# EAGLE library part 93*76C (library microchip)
8K Microwire Compatible Serial EEPROM Source: http://ww1.microchip.com/downloads/en/DeviceDoc/21796H.pdf
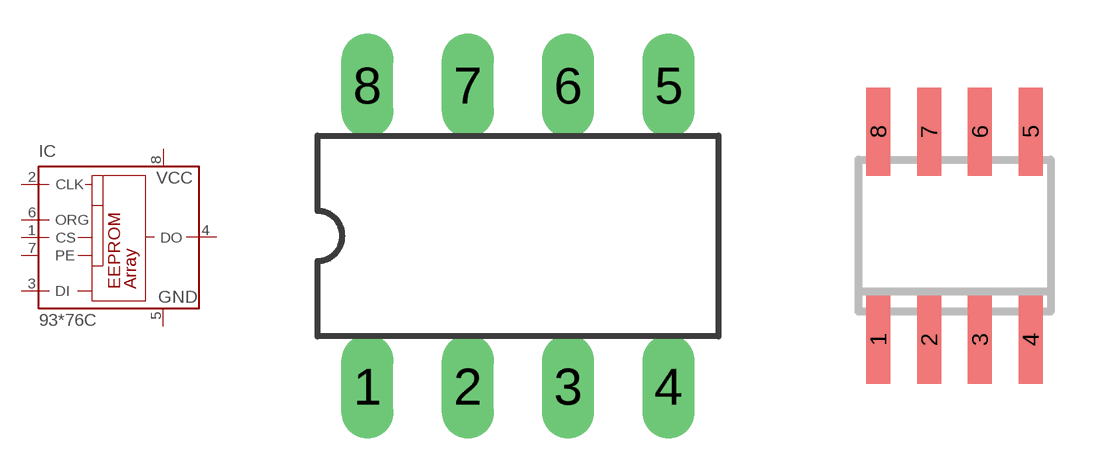
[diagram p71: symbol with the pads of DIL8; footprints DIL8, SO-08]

Designator prefix IC

## 93AA76CP (MF: MICROCHIP; MPN: 93AA76C-I/P; OC_FARNELL: 1331446; OC_NEWARK: 61H6457), 93C76CP (MF: MICROCHIP; MPN: 93C76C-I/P; OC_FARNELL: unknown; OC_NEWARK: 61H6696), 93LC76CP (MPN: 93LC76C-I/P; OC_FARNELL: 1556171; OC_NEWARK: 95M3420)  [DIL8]
1  CS  in
2  CLK  in
3  DI  in
4  DO  hiz
5  GND  pwr
6  ORG  in
7  PE  in
8  VCC  pwr

## 93AA76CSN (MPN: 93AA76C-I/SN; OC_FARNELL: 1331447; OC_NEWARK: 35M2485), 93C76CSN (MF: MICROCHIP; MPN: 93C76C-I/SN; OC_FARNELL: 1815963; OC_NEWARK: 61H6698), 93LC76CSN (MF: MICROCHIP; MPN: 93LC76C-I/SN; OC_FARNELL: unknown; OC_NEWARK: 96K4113)  [SO-08]
Pads as for DIL8

## 93AA76CST (MF: MICROCHIP; MPN: 93AA76CT-I/ST; OC_FARNELL: unknown; OC_NEWARK: 61H6467), 93C76CST (MF: MICROCHIP; MPN: 93C76CT-I/ST; OC_FARNELL: unknown; OC_NEWARK: 61H6709), 93LC76CST (MF: MICROCHIP; MPN: 93LC76C-I/ST; OC_FARNELL: unknown; OC_NEWARK: 96K4114)  [TSSOP8]
Pads as for DIL8

## 93AA76CMS (MPN: 93AA76C-I/MS; OC_FARNELL: 1331445; OC_NEWARK: 35M2483), 93C76CMS (OC_FARNELL: unknown; OC_NEWARK: unknown), 93LC76CMS (MPN: 93LC76C-I/MS; OC_FARNELL: 1331476; OC_NEWARK: 35M2509)  [MSOP8]
Pads as for DIL8

## 9376CMC (OC_FARNELL: unknown; OC_NEWARK: unknown)  [DFN-2X3]
Pads as for DIL8

## Footprint DIL8 (pad centres in mm)
Dual In Line package type P
drill 0.813 long: 1 -3.81,-3.81; 2 -1.27,-3.81; 3 1.27,-3.81; 4 3.81,-3.81; 5 3.81,3.81; 6 1.27,3.81; 7 -1.27,3.81; 8 -3.81,3.81

## Footprint SO-08 (pad centres in mm)
Small Outline Narrow Plastic Gull Wing 150-mil body, package type SN
smd 0.6 x 2.2: 1 -1.905,-2.6; 2 -0.635,-2.6; 3 0.635,-2.6; 4 1.905,-2.6; 5 1.905,2.6; 6 0.635,2.6; 7 -0.635,2.6; 8 -1.905,2.6

## Footprint TSSOP8 (pad centres in mm)
Thin Shrink Small Outline Package package type ST
smd 0.35 x 1.2: 1 -0.975,-2.925; 2 -0.325,-2.925; 3 0.325,-2.925; 4 0.975,-2.925; 5 0.975,2.925; 6 0.325,2.925; 7 -0.325,2.925; 8 -0.975,2.925

## Footprint MSOP8 (pad centres in mm)
Micro Small Outline Package Grid 0.65mm Source: http://ww1.microchip.com/downloads/en/DeviceDoc/21796H.pdf
smd 0.45 x 1: 1 -0.975,-2.05; 2 -0.325,-2.05; 3 0.325,-2.05; 4 0.975,-2.05; 5 0.975,2.05; 6 0.325,2.05; 7 -0.325,2.05; 8 -0.975,2.05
